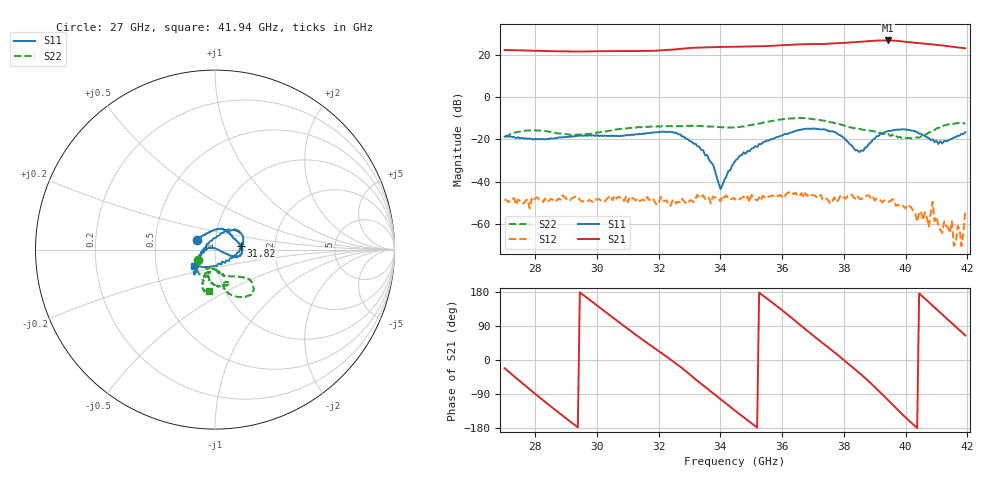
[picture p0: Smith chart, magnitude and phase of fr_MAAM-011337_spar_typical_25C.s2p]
! Created Thu Jan 25 15:57:11 2024
# hz S db R 50
! 2 Port Network Data from SP1.SP block
! freq  dbS11  angS11  dbS21  angS21  dbS12  angS12  dbS22  angS22
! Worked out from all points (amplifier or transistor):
!   240 points, 27 GHz to 41.94 GHz, reference 50 ohm
!   highest |S21| = 26.9 dB at 39.44 GHz (marker M1)
!   |S21| within 3 dB of that: 34.38 GHz to 41.53 GHz (7.153 GHz wide, 18.8 % of centre)
!   unconditionally stable (mu >= 1): start of sweep to end of sweep
!   at 29.5 GHz: K = 11.89, MAG = 21.8 dB, |S12| = -49.4 dB
!   at 34.5 GHz: K = 8.62, MAG = 24.1 dB, |S12| = -48.9 dB
!   at 41.94 GHz: K = 15.97, MAG = 23.5 dB, |S12| = -53.9 dB
!   S11 on the Smith chart (normalised r, x): 27 GHz: 0.81, +0.09; 31.82 GHz: 1.33, +0.05; 41.94 GHz: 0.78, -0.14
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2.70046e10  -18.66 151.6  22.39 -21.7  -48.40 -67.1  -19.01 -148.9
2.806689e10  -19.92 120.4  21.98 -94.1  -47.51 -110.1  -15.88 -112.4
2.95041e10  -18.11 68.3  21.63 174.7  -49.42 -141.5  -17.68 -106.2
3.069136e10  -18.43 34.1  21.86 100.9  -47.21 -178.2  -15.15 -100.6
3.181614e10  -16.78 7.9  21.98 34.2  -48.01 141.4  -14.06 -88.8
3.20036e10  -16.53 4.9  22.11 23.4  -49.94 141.5  -13.76 -86.6
3.281594e10  -18.76 -21.7  23.07 -25.3  -49.29 136.9  -13.65 -75.2
3.356579e10  -27.38 -16.5  23.60 -74.9  -47.39 119.0  -13.91 -67.9
3.45031e10  -29.80 166.0  23.92 -135.4  -48.94 80.8  -14.36 -75.0
3.506549e10  -24.13 -170.6  24.05 -170.6  -47.53 68.9  -12.96 -76.1
3.569036e10  -19.89 -151.3  24.36 150.9  -46.57 48.2  -11.23 -68.8
3.637772e10  -16.40 -132.2  24.94 106.3  -45.89 32.7  -10.03 -54.8
3.70026e10  -14.86 -130.8  25.19 64.5  -46.42 12.4  -10.39 -45.1
3.775245e10  -16.86 -137.9  25.57 16.6  -49.62 -5.9  -12.36 -41.8
3.825235e10  -22.92 -173.3  25.94 -17.4  -46.11 -25.1  -14.40 -51.3
3.893971e10  -20.16 69.7  26.73 -66.4  -46.94 -55.8  -16.03 -70.1
3.943961e10  -16.00 46.1  26.89 -106.3  -49.60 -69.9  -17.49 -80.4
3.95021e10  -16.01 41.1  26.86 -111.6  -49.35 -58.8  -18.42 -80.8
4.0002e10  -15.37 22.8  26.26 -151.8  -52.82 -78.8  -19.37 -98.5
4.05019e10  -17.36 -5.6  25.51 171.4  -54.06 -121.0  -18.63 -113.9
4.125175e10  -20.80 -83.3  24.42 115.5  -58.95 -68.1  -13.36 -110.2
4.193911e10  -16.61 -143.1  23.14 64.6  -53.90 -14.4  -12.64 -98.8
